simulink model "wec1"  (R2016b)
settings: Solver=ode45  StartTime=0  StopTime=1000  FixedStep=0.005  MaxStep=0.005  RelTol=1e-3
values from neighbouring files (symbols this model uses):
  arAdaptiveLawData = 1/2*zModelSimple.zModelPto.arFreq.*     zModelSimple.zModelPto.arMagnitude./     cos(zModelSimple.zModelPto.arPhase*pi/180+pi/2)    [IMPACT_Control.m]
  arControllerRampGain = [0,0,1,1]    [IMPACT_Control.m]
  arControllerRampTime = [0 rStartRampTime rStartRampTime+rRampTimeLength 8000]    [IMPACT_Control.m]
  arEkfInitialisation = zeros(1,11)    [IMPACT_Control.m]
  arFrequency = zModelSimple.zModelPto.arFreq    [IMPACT_Control.m]
  arFrequencyRange = zModelSimple.zModelPto.arFreq    [IMPACT_Control.m]
  arImpedance = 1./zModelSimple.zModelPto.arMagnitude./zModelSimple.zModelPto.arFreq    [IMPACT_Control.m]
  iAdaptiveDamping = 0    [wec1_IMPACT_Project.m]    (also in IMPACT_Control.m = handles.iAdaptiveDamping; wec2_IMPACT_Project.m; wec3_IMPACT_Project.m; wec4IMPACT_Project.m)
  iControlType = 1    [wec1_IMPACT_Project.m]    (also in IMPACT_Control.m = handles.iControlType; wec2_IMPACT_Project.m; wec3_IMPACT_Project.m; wec4IMPACT_Project.m = 2)
  iPtoPositionConstraint = 0    [wec1_IMPACT_Project.m]    (also in IMPACT_Control.m = handles.iPtoPositionConstraint; wec2_IMPACT_Project.m = 1; wec3_IMPACT_Project.m = 1; wec4IMPACT_Project.m = 1)
  iSensorNoise = 0    [IMPACT_Control.m]
  m = m+1    (= 2)    [checkParamFile.m]
  rAccelerationGainPosLim = 9.4530e+06    (= 9453000)    [wec1AdditionalParams.m]    (also in wec2AdditionalParams.m = 4513300)
  rBalancingForce = -(rFloaterVolume*rDENSITY - rFloaterMass)*rGRAVITY    [IMPACT_Control.m]
  rBuoyancyGainPosLim = 3.1355e+06    (= 3135500)    [wec1AdditionalParams.m]    (also in wec2AdditionalParams.m = 7.4216)
  rCogFloater = -18    [wec1_IMPACT_Model.m]    (also in paramInitial.m = get( handles.edit_rCogFloater, 'String' ); wec2_IMPACT_Model.m = -8.5; wec3_IMPACT_Model.m = -0.7; wec3_IMPACT_Model2.m = -0.7)
  rDampingGainPosLim = 2.0369e+05    (= 203690)    [wec1AdditionalParams.m]    (also in wec2AdditionalParams.m = 11575)
  rDisplacementLimit = 10.000000    (= 10)    [wec1_IMPACT_Project.m]    (also in IMPACT_Control.m = getValue(handles.edit_displacementLimit); wec2_IMPACT_Project.m; wec3_IMPACT_Project.m = 3; wec4IMPACT_Project.m)
  rGainForAntiWIndUp = tfControllerDiscrete.rGain    [IMPACT_Control.m]
  rMaxForcePto = 1000000000000000.000000    (= 1e+15)    [wec1_IMPACT_Project.m]    (also in IMPACT_Control.m = getValue(handles.edit_maxForcePto); wec2_IMPACT_Project.m; wec3_IMPACT_Project.m = 1000000000; wec4IMPACT_Project.m = 300000000)
  rMinForcePto = -1000000000000000.000000    (= -1e+15)    [wec1_IMPACT_Project.m]    (also in IMPACT_Control.m = getValue(handles.edit_minForcePto); wec2_IMPACT_Project.m; wec3_IMPACT_Project.m = -1000000000; wec4IMPACT_Project.m = -300000000)
  rOutputSampleTime = 0.010000    (= 0.01)    [wec1_IMPACT_Project.m]    (also in IMPACT_Control.m = getValue(handles.edit_outputSampleTime); wec2_IMPACT_Project.m; wec3_IMPACT_Project.m; wec4IMPACT_Project.m)
  rPassiveDampingGain = -214018.153700    (= -214018.1537)    [wec1_IMPACT_Project.m]    (also in IMPACT_Control.m = getValue(handles.edit_gainPLD); wec2_IMPACT_Project.m = -1948070; wec3_IMPACT_Project.m = -519390; wec4IMPACT_Project.m = -604830)
  rPositionLimitRatio = 10    [wec1AdditionalParams.m]    (also in wec2AdditionalParams.m)
  rUpperFrequencyLimit = EKFFloater.upperFreq    [IMPACT_Control.m]
  s = tf('s')    [wec1_IMPACT_Model.m]    (also in IMPACT_Control.m; wec2_IMPACT_Model.m; wec3_IMPACT_Model.m; wec3_IMPACT_Model2.m)
  simu = simulationClass()    [wecSimInputFile.m]
  Z = magPhaseToComplex(zModelTf)    [IMPACT_Control.m]
undefined symbols (not defined in the file or in its folder): arExcForceFloaterDen, arExcForceFloaterNum, body, N, pto, rAccelerationGainFloater, rBuoyancyGainFloater, rDampingGainFloater, X, Y
libraries: nesl_utility x9, sm_lib x5, simulink x3, WECSim_Lib x2

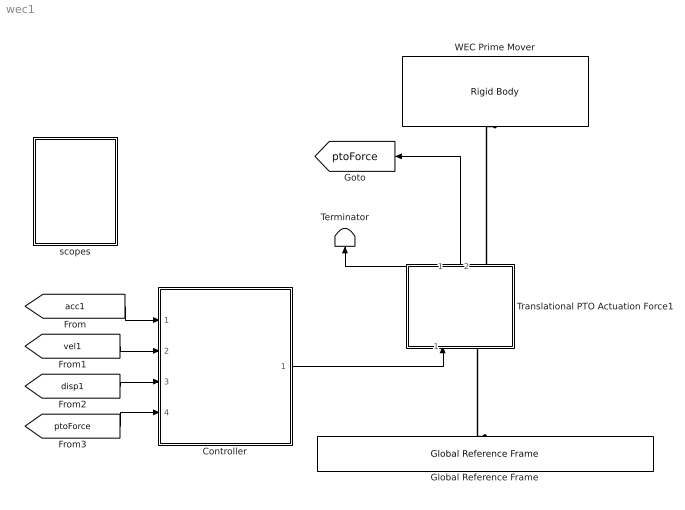
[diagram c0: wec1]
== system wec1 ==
  Controller : Subsystem
  Global Reference Frame : WECSim_Lib/Frames/Global Reference Frame  waves=waves  simu=simu
  Terminator : Terminator
  Translational PTO Actuation Force1 : Subsystem  AncestorBlock=WECSim_Lib/PTOs/Translational PTO Actuation Force
  WEC Prime Mover : WECSim_Lib/Body Elements/Rigid Body  body=body(1)
  scopes : Subsystem
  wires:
  Translational PTO Actuation Force1/2(ptoForce) -> [ptoForce]
  Controller/1(forceDemand) -> Translational PTO Actuation Force1/1(Force)
  Translational PTO Actuation Force1/1(Response) -> Terminator/1
  [disp1] -> Controller/3(Floater displacement)
  [vel1] -> Controller/2(Floater velocity)
  [acc1] -> Controller/1(Floater acceleration)
  [ptoForce] -> Controller/4(PTO Force)
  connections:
  Translational PTO Actuation Force1/RConn1 -- WEC Prime Mover/RConn1
  Translational PTO Actuation Force1/LConn1 -- Global Reference Frame/RConn1

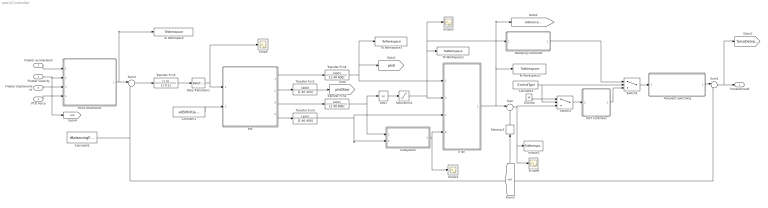
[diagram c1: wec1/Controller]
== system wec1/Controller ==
  Floater acceleration : Inport
  Floater velocity : Inport  Port=2
  Floater displacement : Inport  Port=3
  PTO Force : Inport  Port=4
  Abs1 : Abs
  Constant1 : Constant  Value=arEkfInitialisation
  Constant3 : Constant  Value=iControlType
  Constant5 : Constant  Value=rBalancingForce
  Damping Controller : Subsystem
  EKF : MATLAB Function  TreatAsAtomicUnit=on
  "Force estimation " : Subsystem
  Ground : Ground
  OVT Controller : Subsystem
  Rate Transition1 : RateTransition  OutPortSampleTimeMultiple=0.01  OutPortSampleTime=rKalmanFilterSampleTime
  Saturation1 : Saturate  UpperLimit=rUpperFrequencyLimit  LowerLimit=0  LinearizeAsGain=off
  Scope{,1..2,8} (4 alike) : Scope
  Selector2 : Selector  InputPortWidth=6  IndexOptions=Index vector (dialog)  Indices=3  OutputSizes=1
  Subsystem : Subsystem
  Sum : Sum  Inputs=|+-
  Sum1 : Sum  Inputs=|++
  Sum2 : Sum  Inputs=|++
  Switch1 : Switch  Threshold=2
  Switch2 : Switch  Threshold=2
  To Workspace : ToWorkspace  VariableName=arEstimatedExcitationForce1  SampleTime=rOutputSampleTime
  To Workspace1 : ToWorkspace  VariableName=arEkfFrequency  SampleTime=rOutputSampleTime
  To Workspace2 : ToWorkspace  VariableName=arReferenceVelocity  SampleTime=rOutputSampleTime
  To Workspace3 : ToWorkspace  VariableName=arEkfAmplitude  SampleTime=rOutputSampleTime
  Transfer Fcn{1..2,4..5} (4 alike) : TransferFcn  Numerator=[400]  Denominator=[1 40 400]
  Transfer Fcn3 : TransferFcn  Numerator=[1 0]  Denominator=[1 0.1]
  Transient Switching : Subsystem
  "V ref " : Subsystem
  output1 : ToWorkspace  VariableName=arError  SampleTime=rOutputSampleTime
  forceDemand : Outport
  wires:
  Damping Controller/1(forceDemand) -> Switch1/1
  Sum/1 -> output1/1, Scope8/1, Switch2/3
  Selector2/1 -> Sum/2
  "V ref "/1(referenceVelocity) -> To Workspace2/1, [referenceVelocity], Sum/1
  [vel1] -> Selector2/1
  OVT Controller/1(forceDemand) -> Switch1/3
  Saturation1/1 -> Scope2/1, Damping Controller/1(ekfFrequency), To Workspace1/1, "V ref "/2(ekfFrequency)
  EKF/4(rAmplitudeOutput) -> Transfer Fcn5/1
  EKF/3(rFrequencyOutput) -> Transfer Fcn2/1
  EKF/1(rPhi0Output) -> Transfer Fcn4/1
  Rate Transition1/1 -> Scope/1, EKF/1(rEstimatedExcitationForce)
  EKF/2(rPhi0StarOutput) -> Transfer Fcn1/1
  Abs1/1 -> Saturation1/1
  Switch1/1 -> Transient Switching/1(forceDemandIn)
  Sum1/1 -> [forceDemand], forceDemand/1
  Constant5/1 -> Sum1/2, Sum2/2
  Transfer Fcn3/1 -> Rate Transition1/1
  Constant1/1 -> EKF/2(arEkfInitialisation)
  "Force estimation "/1(estimatedExcitationForce) -> To Workspace/1, Sum2/1
  Switch2/1 -> OVT Controller/1(error)
  Transient Switching/1(forceDemandOut) -> Sum1/1
  Sum2/1 -> Transfer Fcn3/1
  Transfer Fcn4/1 -> "V ref "/1(phiOut), To Workspace3/1, [phi0]
  Transfer Fcn1/1 -> [phi0Star]
  Transfer Fcn2/1 -> Abs1/1, Subsystem/1(frequency)
  Transfer Fcn5/1 -> Subsystem/2(excitationForce), "V ref "/3(ekfAmplitude)
  Subsystem/1(displacementLimit) -> Scope1/1, "V ref "/4(limit)
  Ground/1 -> Switch2/1
  Floater acceleration/1 -> "Force estimation "/1(Acceleration)
  Floater displacement/1 -> "Force estimation "/3(Position)
  Floater velocity/1 -> [vel1], "Force estimation "/2(Velocity)
  PTO Force/1 -> "Force estimation "/4(PTO Force)
  Constant3/1 -> Switch2/2, Switch1/2

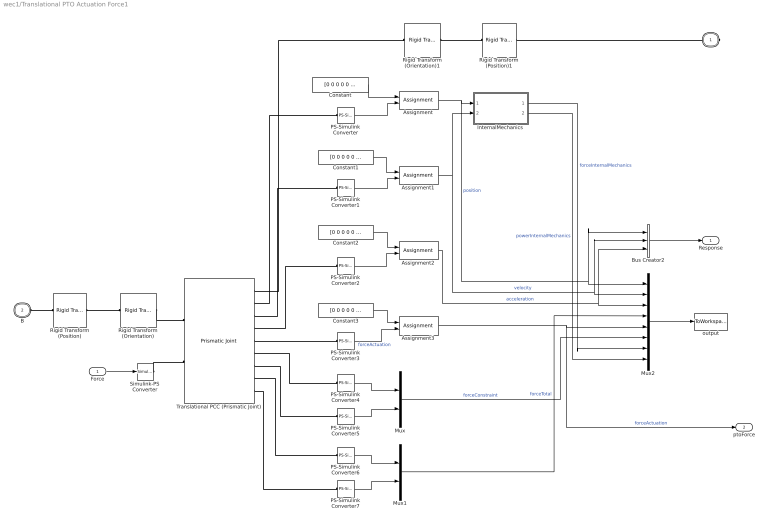
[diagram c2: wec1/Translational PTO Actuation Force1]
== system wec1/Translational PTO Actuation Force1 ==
  Force : Inport
  Assignment{,1..3} (4 alike) : Assignment  IndexOptions=Index vector (dialog)  Indices=3  OutputSizes=1
  Bus Creator2 : BusCreator  Inputs=3
  Constant{,1..3} (4 alike) : Constant  Value=[0 0 0 0 0 0]
  InternalMechanics : Subsystem
  Mux : Mux  Inputs=2
  Mux1 : Mux  Inputs=2
  Mux2 : Mux  Inputs=8
  PS-Simulink Converter{,1..7} (8 alike) : nesl_utility/PS-Simulink Converter  PhysicalDomain=network_engine_domain  SubClassName=ps_output  LeftPortType=input  RightPortType=output  PseudoPeriodic=off  Frequencies=[]  Unit=1  AffineConversion=off
  Rigid Transform (Position) : sm_lib/Frames and Transforms/Rigid Transform  TranslationMethod=Cartesian  TranslationStandardOffset=0  TranslationLengthUnit=m  TranslationStandardAxis=+Z  TranslationCartesianOffset=pto.initDisp.initLinDisp + pto.loc  TranslationROffset=0  TranslationROffsetUnits=m  TranslationZOffset=0  TranslationZOffsetUnits=m  TranslationThetaOffset=0  TranslationThetaOffsetUnits=deg  RotationMethod=None  RotationAngleUnits=rad  RotationStandardAxis=+Y  RotationAngle=0  RotationArbitraryAxis=[0 1 0]  FollAlignAxisA=+X  BaseAlignAxisA=+Y  FollAlignAxisB=+Y  BaseAlignAxisB=+Z  RotationSequenceAxes=FollowerAxes  RotationSequence=XYX  RotationSequenceAngles=[0 0 0]  RotationSequenceAnglesUnits=deg  RotationMatrix=[1 0 0; 0 1 0; 0 0 1]
  Rigid Transform (Position)1 : sm_lib/Frames and Transforms/Rigid Transform  TranslationMethod=Cartesian  TranslationStandardOffset=0  TranslationLengthUnit=m  TranslationStandardAxis=+Z  TranslationCartesianOffset=pto.initDisp.initLinDisp + pto.loc  TranslationROffset=0  TranslationROffsetUnits=m  TranslationZOffset=0  TranslationZOffsetUnits=m  TranslationThetaOffset=0  TranslationThetaOffsetUnits=deg  RotationMethod=None  RotationAngleUnits=rad  RotationStandardAxis=+Y  RotationAngle=0  RotationArbitraryAxis=[0 1 0]  FollAlignAxisA=+X  BaseAlignAxisA=+Y  FollAlignAxisB=+Y  BaseAlignAxisB=+Z  RotationSequenceAxes=FollowerAxes  RotationSequence=XYX  RotationSequenceAngles=[0 0 0]  RotationSequenceAnglesUnits=deg  RotationMatrix=[1 0 0; 0 1 0; 0 0 1]
  Rigid Transform (Orientation) : sm_lib/Frames and Transforms/Rigid Transform  TranslationMethod=None  TranslationStandardOffset=0  TranslationLengthUnit=m  TranslationStandardAxis=+Z  TranslationCartesianOffset=0  TranslationROffset=0  TranslationROffsetUnits=m  TranslationZOffset=0  TranslationZOffsetUnits=m  TranslationThetaOffset=0  TranslationThetaOffsetUnits=deg  RotationMethod=RotationMatrix  RotationAngleUnits=rad  RotationStandardAxis=+Y  RotationAngle=0  RotationArbitraryAxis=[0 1 0]  FollAlignAxisA=+X  BaseAlignAxisA=+Y  FollAlignAxisB=+Y  BaseAlignAxisB=+Z  RotationSequenceAxes=FollowerAxes  RotationSequence=XYX  RotationSequenceAngles=[0 0 0]  RotationSequenceAnglesUnits=deg  RotationMatrix=pto.orientation.rotationMatrix
  Rigid Transform (Orientation)1 : sm_lib/Frames and Transforms/Rigid Transform  TranslationMethod=None  TranslationStandardOffset=0  TranslationLengthUnit=m  TranslationStandardAxis=+Z  TranslationCartesianOffset=0  TranslationROffset=0  TranslationROffsetUnits=m  TranslationZOffset=0  TranslationZOffsetUnits=m  TranslationThetaOffset=0  TranslationThetaOffsetUnits=deg  RotationMethod=RotationMatrix  RotationAngleUnits=rad  RotationStandardAxis=+Y  RotationAngle=0  RotationArbitraryAxis=[0 1 0]  FollAlignAxisA=+X  BaseAlignAxisA=+Y  FollAlignAxisB=+Y  BaseAlignAxisB=+Z  RotationSequenceAxes=FollowerAxes  RotationSequence=XYX  RotationSequenceAngles=[0 0 0]  RotationSequenceAnglesUnits=deg  RotationMatrix=pto.orientation.rotationMatrix
  Simulink-PS Converter : nesl_utility/Simulink-PS Converter  PhysicalDomain=network_engine_domain  SubClassName=ps_input  LeftPortType=input  RightPortType=output  PseudoPeriodic=off  Frequencies=[]  NoiseDistribution=none  NoiseParameters=[]  Unit=1  AffineConversion=off  InputFiltering=off  SimscapeFilterOrder=1  InputFilterTimeConstant=0.001  UdotUserProvided=1
  Translational PCC (Prismatic Joint) : sm_lib/Joints/Prismatic Joint  SenseConstraintForce=on  SenseConstraintForceX=off  SenseConstraintForceY=off  SenseConstraintForceZ=off  SenseConstraintTorque=on  SenseConstraintTorqueX=off  SenseConstraintTorqueY=off  SenseConstraintTorqueZ=off  SenseTotalForce=on  SenseTotalForceX=off  SenseTotalForceY=off  SenseTotalForceZ=off  SenseTotalTorque=on  SenseTotalTorqueX=off  SenseTotalTorqueY=off  SenseTotalTorqueZ=off  CompositeWrenchDir=BaseOnFollower  CompositeWrenchFrame=BaseFrame  EquilibriumPosition=0  EquilibriumPositionUnits=m  SpringStiffness=pto.k  SpringStiffnessUnits=N/m  DampingCoefficient=pto.c  DampingCoefficientUnits=N/(m/s)  TorqueActuationMode=InputTorque  MotionActuationMode=ComputedMotion  SensePosition=on  SenseVelocity=on  SenseAcceleration=on  SenseTorqueForce=on  PositionTargetSpecify=off  PositionTargetPriority=High  PositionTargetValue=0  PositionTargetValueUnits=m  VelocityTargetSpecify=off  VelocityTargetPriority=High  VelocityTargetValue=0  VelocityTargetValueUnits=m/s
  output : ToWorkspace  VariableName=pto1_out  SaveFormat=Structure With Time  SampleTime=-1
  F : PMIOPort  Port=1  Side=Right
  B : PMIOPort  Port=2  Side=Left
  Response : Outport
  ptoForce : Outport  Port=2
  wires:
  Bus Creator2/1 -> Response/1
  Assignment/1 -> Mux2/1, Bus Creator2/1, InternalMechanics/1(Position)  "position"
  Assignment1/1 -> Mux2/2, Bus Creator2/2, InternalMechanics/2(Velocity)  "velocity"
  Assignment2/1 -> Mux2/3, Bus Creator2/3  "acceleration"
  Force/1 -> Simulink-PS Converter/1
  Mux2/1 -> output/1
  Mux/1 -> Mux2/6  "forceConstraint"
  Mux1/1 -> Mux2/4  "forceTotal"
  PS-Simulink Converter4/1 -> Mux/1
  PS-Simulink Converter5/1 -> Mux/2
  PS-Simulink Converter6/1 -> Mux1/1
  PS-Simulink Converter7/1 -> Mux1/2
  Assignment3/1 -> ptoForce/1, Mux2/5  "forceActuation"
  Constant/1 -> Assignment/1
  PS-Simulink Converter/1 -> Assignment/2
  Constant1/1 -> Assignment1/1
  PS-Simulink Converter1/1 -> Assignment1/2
  Constant2/1 -> Assignment2/1
  PS-Simulink Converter2/1 -> Assignment2/2
  InternalMechanics/1(Force) -> Mux2/7  "forceInternalMechanics"
  InternalMechanics/2(Power) -> Mux2/8  "powerInternalMechanics"
  Constant3/1 -> Assignment3/1
  PS-Simulink Converter3/1 -> Assignment3/2  "forceActuation"
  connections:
  Rigid Transform (Position)/RConn1 -- Rigid Transform (Orientation)/LConn1
  Rigid Transform (Position)1/RConn1 -- Rigid Transform (Orientation)1/LConn1
  Simulink-PS Converter/RConn1 -- Translational PCC (Prismatic Joint)/LConn2
  Rigid Transform (Orientation)/RConn1 -- Translational PCC (Prismatic Joint)/LConn1
  Rigid Transform (Position)/LConn1 -- B/RConn1
  Translational PCC (Prismatic Joint)/RConn5 -- PS-Simulink Converter3/LConn1
  Translational PCC (Prismatic Joint)/RConn9 -- PS-Simulink Converter7/LConn1
  Rigid Transform (Orientation)1/RConn1 -- Translational PCC (Prismatic Joint)/RConn1
  Translational PCC (Prismatic Joint)/RConn4 -- PS-Simulink Converter2/LConn1
  Translational PCC (Prismatic Joint)/RConn7 -- PS-Simulink Converter5/LConn1
  Translational PCC (Prismatic Joint)/RConn3 -- PS-Simulink Converter1/LConn1
  Rigid Transform (Position)1/LConn1 -- F/RConn1
  Translational PCC (Prismatic Joint)/RConn8 -- PS-Simulink Converter6/LConn1
  Translational PCC (Prismatic Joint)/RConn2 -- PS-Simulink Converter/LConn1
  Translational PCC (Prismatic Joint)/RConn6 -- PS-Simulink Converter4/LConn1

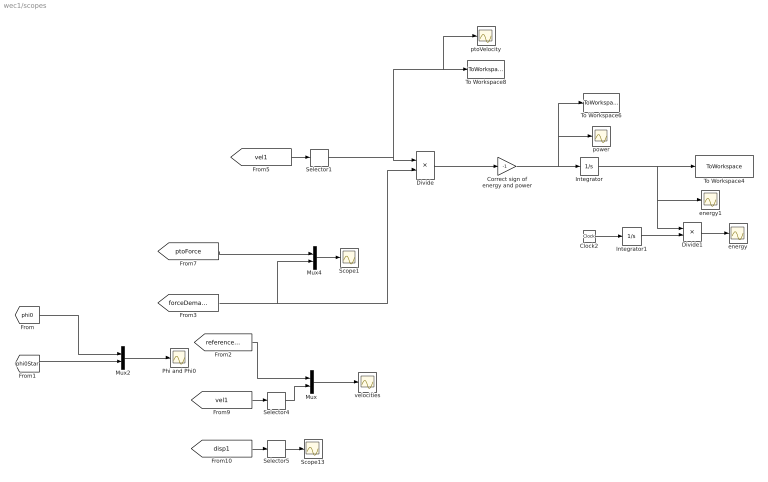
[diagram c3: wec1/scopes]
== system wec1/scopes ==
  Clock2 : Clock
  Correct sign of energy and power : Gain  Gain=-1
  Divide : Product  Inputs=**
  Divide1 : Product  Inputs=*/
  Integrator : Integrator
  Integrator1 : Integrator
  Mux : Mux  Inputs=2
  Mux2 : Mux  Inputs=2
  Mux4 : Mux  Inputs=2
  Phi and Phi0 : Scope
  Scope1 : Scope
  Scope13 : Scope
  Selector1 : Selector  InputPortWidth=6  IndexOptions=Index vector (dialog)  Indices=3  OutputSizes=1
  Selector4 : Selector  InputPortWidth=6  IndexOptions=Index vector (dialog)  Indices=3  OutputSizes=1
  Selector5 : Selector  InputPortWidth=6  IndexOptions=Index vector (dialog)  Indices=3  OutputSizes=1
  To Workspace4 : ToWorkspace  VariableName=arWecEnergy  SampleTime=rOutputSampleTime
  To Workspace6 : ToWorkspace  VariableName=arWecPower  SampleTime=rOutputSampleTime
  To Workspace8 : ToWorkspace  VariableName=arPtoVelocity  SampleTime=rOutputSampleTime
  energy : Scope
  energy1 : Scope
  power : Scope
  ptoVelocity : Scope
  velocities : Scope
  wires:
  [vel1] -> Selector4/1
  Mux/1 -> velocities/1
  Selector5/1 -> Scope13/1
  [phi0] -> Mux2/1
  Mux2/1 -> Phi and Phi0/1
  Mux4/1 -> Scope1/1
  Selector4/1 -> Mux/2
  [disp1] -> Selector5/1
  [referenceVelocity] -> Mux/1
  [forceDemand] -> Mux4/2, Divide/2
  Clock2/1 -> Integrator1/1
  Divide1/1 -> energy/1
  Integrator1/1 -> Divide1/2
  Integrator/1 -> To Workspace4/1, energy1/1, Divide1/1
  Divide/1 -> Correct sign of energy and power/1
  Selector1/1 -> Divide/1, ptoVelocity/1, To Workspace8/1
  [vel1] -> Selector1/1
  [phi0Star] -> Mux2/2
  Correct sign of energy and power/1 -> To Workspace6/1, power/1, Integrator/1
  [ptoForce] -> Mux4/1

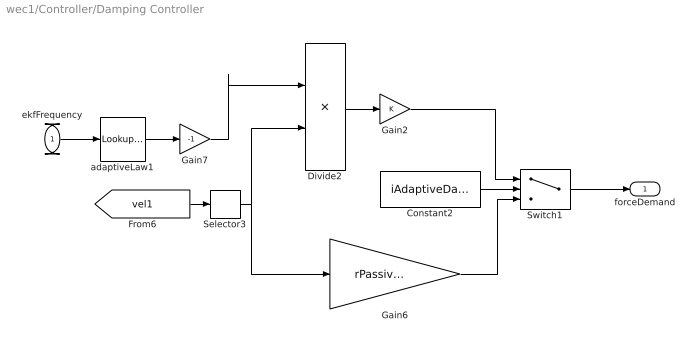
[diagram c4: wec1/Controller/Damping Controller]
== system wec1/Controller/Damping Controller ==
  ekfFrequency : Inport
  Constant2 : Constant  Value=iAdaptiveDamping
  Divide2 : Product  Inputs=**
  Gain2 : Gain
  Gain6 : Gain  Gain=rPassiveDampingGain
  Gain7 : Gain  Gain=-1
  Selector3 : Selector  InputPortWidth=6  IndexOptions=Index vector (dialog)  Indices=3  OutputSizes=1
  Switch1 : Switch  Criteria=u2 > Threshold
  adaptiveLaw1 : Lookup_n-D  NumberOfTableDimensions=1  BreakpointsForDimension1=arFrequency  Table=arImpedance  InternalRulePriority=Speed  RndMeth=Simplest
  forceDemand : Outport
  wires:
  Gain2/1 -> Switch1/1
  ekfFrequency/1 -> adaptiveLaw1/1
  adaptiveLaw1/1 -> Gain7/1
  Constant2/1 -> Switch1/2
  Switch1/1 -> forceDemand/1
  Gain7/1 -> Divide2/1
  Selector3/1 -> Divide2/2, Gain6/1
  [vel1] -> Selector3/1
  Divide2/1 -> Gain2/1
  Gain6/1 -> Switch1/3

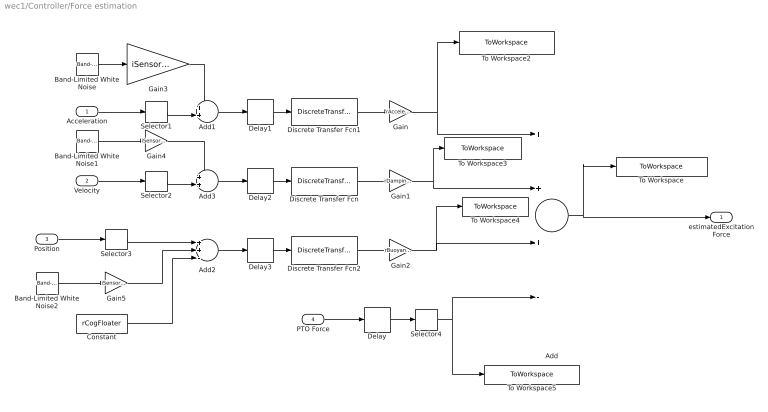
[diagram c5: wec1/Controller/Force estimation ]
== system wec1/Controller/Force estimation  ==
  Acceleration : Inport
  Velocity : Inport  Port=2
  Position : Inport  Port=3
  PTO Force : Inport  Port=4
  Add : Sum  Inputs=+++-
  Add1 : Sum  Inputs=++|
  Add2 : Sum  Inputs=++-
  Add3 : Sum  Inputs=++|
  Band-Limited White Noise : simulink/Sources/Band-Limited White Noise  Cov=rAccNoisePower  Ts=simu.dt  seed=[23341]
  Band-Limited White Noise1 : simulink/Sources/Band-Limited White Noise  Cov=rVelNoisePower  Ts=simu.dt  seed=[23341]
  Band-Limited White Noise2 : simulink/Sources/Band-Limited White Noise  Cov=rPosNoisePower  Ts=simu.dt  seed=[23341]
  Constant : Constant  Value=rCogFloater
  Delay{,1..3} (4 alike) : Delay  DelayLength=1  SampleTime=0.01
  Discrete Transfer Fcn : DiscreteTransferFcn  Numerator=arExcForceFloaterNum  Denominator=arExcForceFloaterDen  SampleTime=0.01
  Discrete Transfer Fcn1 : DiscreteTransferFcn  Numerator=arExcForceFloaterNum  Denominator=arExcForceFloaterDen  SampleTime=0.01
  Discrete Transfer Fcn2 : DiscreteTransferFcn  Numerator=arExcForceFloaterNum  Denominator=arExcForceFloaterDen  SampleTime=0.01
  Gain : Gain  Gain=rAccelerationGainFloater
  Gain1 : Gain  Gain=rDampingGainFloater
  Gain2 : Gain  Gain=rBuoyancyGainFloater
  Gain3 : Gain  Gain=iSensorNoise
  Gain4 : Gain  Gain=iSensorNoise
  Gain5 : Gain  Gain=iSensorNoise
  Selector{1..4} (4 alike) : Selector  InputPortWidth=6  IndexOptions=Index vector (dialog)  Indices=3  OutputSizes=1
  To Workspace : ToWorkspace  VariableName=arEstimatedExcitationForce  SampleTime=rOutputSampleTime
  To Workspace2 : ToWorkspace  VariableName=arAccelerationComponent  SampleTime=rOutputSampleTime
  To Workspace3 : ToWorkspace  VariableName=arVelocityComponent  SampleTime=rOutputSampleTime
  To Workspace4 : ToWorkspace  VariableName=arPositionComponent  SampleTime=rOutputSampleTime
  To Workspace5 : ToWorkspace  VariableName=arPtoForceMeasurement  SampleTime=rOutputSampleTime
  estimatedExcitationForce : Outport
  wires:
  Selector1/1 -> Add1/2
  Band-Limited White Noise/1 -> Gain3/1
  Acceleration/1 -> Selector1/1
  Gain5/1 -> Add2/2
  Add2/1 -> Delay3/1
  Position/1 -> Selector3/1
  Add/1 -> To Workspace/1, estimatedExcitationForce/1
  Gain2/1 -> To Workspace4/1, Add/3
  Gain/1 -> To Workspace2/1, Add/1
  Constant/1 -> Add2/3
  Gain4/1 -> Add3/1
  Velocity/1 -> Selector2/1
  Gain3/1 -> Add1/1
  Selector2/1 -> Add3/2
  Add1/1 -> Delay1/1
  Selector3/1 -> Add2/1
  Band-Limited White Noise1/1 -> Gain4/1
  Band-Limited White Noise2/1 -> Gain5/1
  Selector4/1 -> To Workspace5/1, Add/4
  Delay/1 -> Selector4/1
  Delay1/1 -> Discrete Transfer Fcn1/1
  Delay2/1 -> Discrete Transfer Fcn/1
  Delay3/1 -> Discrete Transfer Fcn2/1
  Gain1/1 -> Add/2, To Workspace3/1
  Add3/1 -> Delay2/1
  Discrete Transfer Fcn1/1 -> Gain/1
  Discrete Transfer Fcn/1 -> Gain1/1
  Discrete Transfer Fcn2/1 -> Gain2/1
  PTO Force/1 -> Delay/1

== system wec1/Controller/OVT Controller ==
  error : Inport
  Anti wind-up controller : Subsystem
  forceDemand : Outport
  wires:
  error/1 -> Anti wind-up controller/1(error)
  Anti wind-up controller/1(Out1) -> forceDemand/1

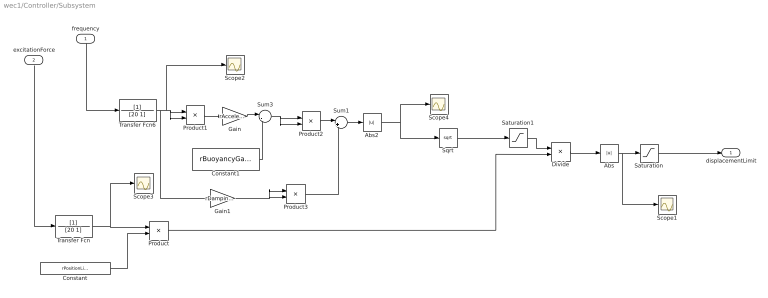
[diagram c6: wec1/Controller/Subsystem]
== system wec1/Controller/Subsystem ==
  frequency : Inport
  excitationForce : Inport  Port=2
  Abs : Abs
  Abs2 : Abs
  Constant : Constant  Value=rPositionLimitRatio
  Constant1 : Constant  Value=rBuoyancyGainPosLim
  Divide : Product  Inputs=/*
  Gain : Gain  Gain=rAccelerationGainPosLim
  Gain1 : Gain  Gain=rDampingGainPosLim
  Product{,1..3} (4 alike) : Product
  Saturation : Saturate  UpperLimit=10  LowerLimit=0
  Saturation1 : Saturate  UpperLimit=inf  LowerLimit=0.0001
  Scope{1..4} (4 alike) : Scope
  Sqrt : Sqrt
  Sum1 : Sum  Inputs=|++
  Sum3 : Sum  Inputs=|-+
  Transfer Fcn : TransferFcn  Denominator=[20 1]
  Transfer Fcn6 : TransferFcn  Denominator=[20 1]
  displacementLimit : Outport
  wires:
  Product1/1 -> Gain/1
  Gain/1 -> Sum3/1
  Transfer Fcn6/1 -> Gain1/1, Scope2/1, Product1/2, Product1/1
  Constant1/1 -> Sum3/2
  Product/1 -> Divide/2
  Constant/1 -> Product/2
  Transfer Fcn/1 -> Scope3/1, Product/1
  frequency/1 -> Transfer Fcn6/1
  excitationForce/1 -> Transfer Fcn/1
  Divide/1 -> Abs/1
  Sum3/1 -> Product2/1, Product2/2
  Abs/1 -> Scope1/1, Saturation/1
  Saturation/1 -> displacementLimit/1
  Saturation1/1 -> Divide/1
  Abs2/1 -> Scope4/1, Sqrt/1
  Product2/1 -> Sum1/1
  Gain1/1 -> Product3/1, Product3/2
  Product3/1 -> Sum1/2
  Sum1/1 -> Abs2/1
  Sqrt/1 -> Saturation1/1

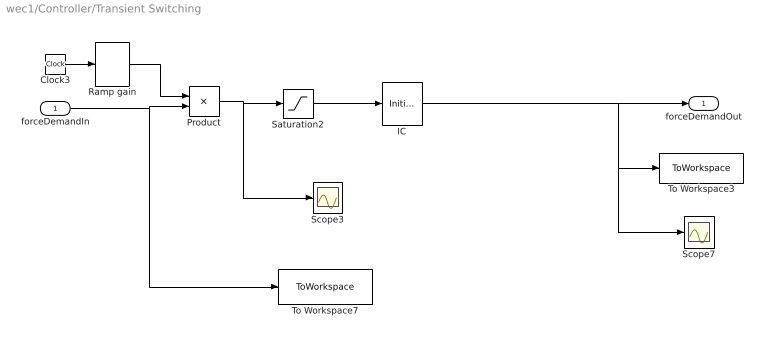
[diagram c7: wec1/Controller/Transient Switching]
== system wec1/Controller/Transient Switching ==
  forceDemandIn : Inport
  Clock3 : Clock
  IC : InitialCondition  Value=0
  Product : Product
  Ramp gain : Lookup_n-D  NumberOfTableDimensions=1  BreakpointsForDimension1=arControllerRampTime  Table=arControllerRampGain  InternalRulePriority=Speed  RndMeth=Simplest
  Saturation2 : Saturate  UpperLimit=rMaxForcePto  LowerLimit=rMinForcePto
  Scope3 : Scope
  Scope7 : Scope
  To Workspace3 : ToWorkspace  VariableName=arForceDemand  SampleTime=rOutputSampleTime
  To Workspace7 : ToWorkspace  VariableName=arForceDemandIn  SampleTime=rOutputSampleTime
  forceDemandOut : Outport
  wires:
  Clock3/1 -> Ramp gain/1
  Saturation2/1 -> IC/1
  Product/1 -> Saturation2/1, Scope3/1
  forceDemandIn/1 -> Product/2, To Workspace7/1
  IC/1 -> To Workspace3/1, Scope7/1, forceDemandOut/1
  Ramp gain/1 -> Product/1

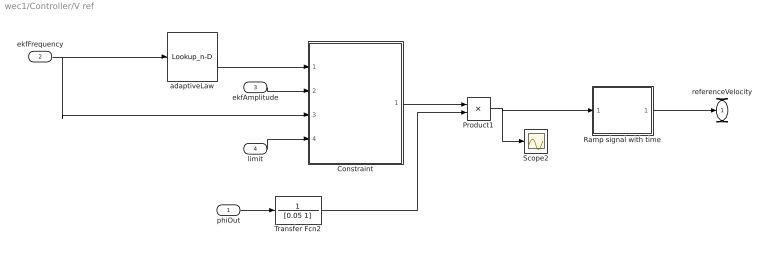
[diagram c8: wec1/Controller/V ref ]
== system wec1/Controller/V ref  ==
  phiOut : Inport
  ekfFrequency : Inport  Port=2
  ekfAmplitude : Inport  Port=3
  limit : Inport  Port=4
  Constraint : Subsystem
  Product1 : Product
  Ramp signal with time : Subsystem
  Scope2 : Scope
  Transfer Fcn2 : TransferFcn  Numerator=1  Denominator=[0.05 1]
  adaptiveLaw : Lookup_n-D  NumberOfTableDimensions=1  BreakpointsForDimension1=arFrequencyRange  Table=arAdaptiveLawData  InternalRulePriority=Speed  RndMeth=Simplest
  referenceVelocity : Outport
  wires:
  Constraint/1(referenceVelocity) -> Product1/1
  phiOut/1 -> Transfer Fcn2/1
  adaptiveLaw/1 -> Constraint/1(1/2B)
  ekfFrequency/1 -> Constraint/3(ekfFrequency), adaptiveLaw/1
  Transfer Fcn2/1 -> Product1/2
  ekfAmplitude/1 -> Constraint/2(Amp)
  Product1/1 -> Ramp signal with time/1(In1), Scope2/1
  limit/1 -> Constraint/4(limit)
  Ramp signal with time/1(Out1) -> referenceVelocity/1

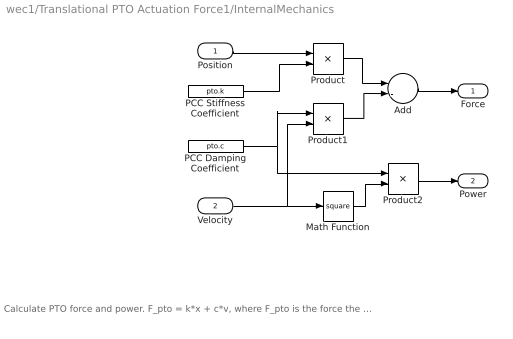
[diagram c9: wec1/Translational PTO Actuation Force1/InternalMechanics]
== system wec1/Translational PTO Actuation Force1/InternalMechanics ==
  note: Calculate PTO force and power. F_pto = k*x + c*v, where F_pto is the force the PTO applies to the body (at the PTO location), x and v are the joint position and velocity. The power extracted is P = c * v^2
  Position : Inport
  Velocity : Inport  Port=2
  Add : Sum  Inputs=--
  Math Function : Math  Operator=square
  PCC Damping Coefficient : Constant  Value=pto.c
  PCC Stiffness Coefficient : Constant  Value=pto.k
  Product : Product  Inputs=**
  Product1 : Product  Inputs=**
  Product2 : Product  Inputs=**
  Force : Outport
  Power : Outport  Port=2
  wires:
  PCC Damping Coefficient/1 -> Product2/1, Product1/1
  Product2/1 -> Power/1
  Velocity/1 -> Math Function/1, Product1/2
  PCC Stiffness Coefficient/1 -> Product/2
  Position/1 -> Product/1
  Add/1 -> Force/1
  Math Function/1 -> Product2/2
  Product/1 -> Add/1
  Product1/1 -> Add/2

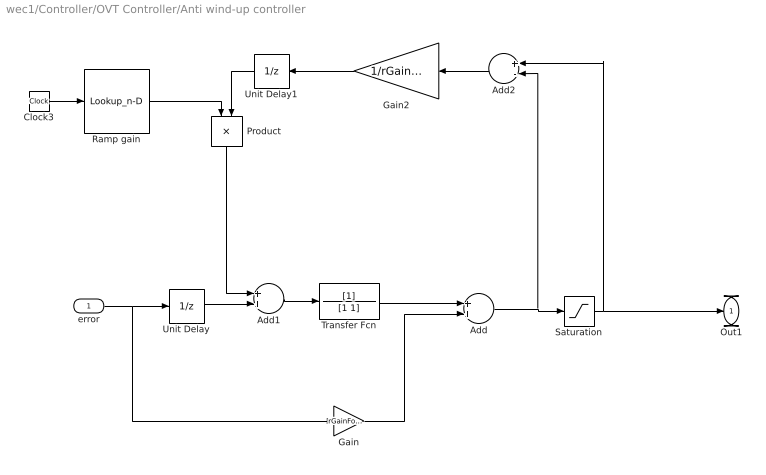
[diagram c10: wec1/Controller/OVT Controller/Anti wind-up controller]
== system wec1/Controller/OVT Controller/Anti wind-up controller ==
  error : Inport
  Add : Sum
  Add1 : Sum
  Add2 : Sum  Inputs=+-
  Clock3 : Clock
  Gain : Gain  Gain=rGainForAntiWIndUp
  Gain2 : Gain  Gain=1/rGainForAntiWIndUp
  Product : Product
  Ramp gain : Lookup_n-D  NumberOfTableDimensions=1  BreakpointsForDimension1=arControllerRampTime  Table=arControllerRampGain  InternalRulePriority=Speed  RndMeth=Simplest
  Saturation : Saturate  UpperLimit=rMaxForcePto  LowerLimit=rMinForcePto
  Transfer Fcn : TransferFcn  Denominator=[1 1]
  Unit Delay : UnitDelay  SampleTime=0.01
  Unit Delay1 : UnitDelay  SampleTime=0.01
  Out1 : Outport
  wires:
  Add/1 -> Saturation/1, Add2/2
  Gain/1 -> Add/2
  Unit Delay/1 -> Add1/2
  Gain2/1 -> Unit Delay1/1
  error/1 -> Gain/1, Unit Delay/1
  Add2/1 -> Gain2/1
  Add1/1 -> Transfer Fcn/1
  Clock3/1 -> Ramp gain/1
  Ramp gain/1 -> Product/1
  Product/1 -> Add1/1
  Unit Delay1/1 -> Product/2
  Transfer Fcn/1 -> Add/1
  Saturation/1 -> Add2/1, Out1/1

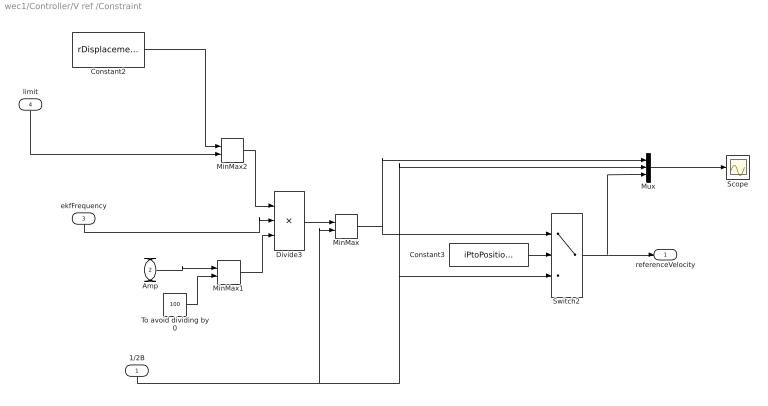
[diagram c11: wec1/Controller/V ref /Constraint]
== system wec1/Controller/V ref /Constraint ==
  1/2B : Inport
  Amp : Inport  Port=2
  ekfFrequency : Inport  Port=3
  limit : Inport  Port=4
  Constant2 : Constant  Value=rDisplacementLimit
  Constant3 : Constant  Value=iPtoPositionConstraint
  Divide3 : Product  Inputs=**/
  MinMax : MinMax  Inputs=2
  MinMax1 : MinMax  Function=max  Inputs=2
  MinMax2 : MinMax  Inputs=2
  Mux : Mux  Inputs=3
  Scope : Scope
  Switch2 : Switch  Criteria=u2 > Threshold
  To avoid dividing by 0 : Constant  Value=100
  referenceVelocity : Outport
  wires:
  MinMax/1 -> Mux/1, Switch2/1
  ekfFrequency/1 -> Divide3/2
  limit/1 -> MinMax2/2
  MinMax1/1 -> Divide3/3
  Divide3/1 -> MinMax/1
  To avoid dividing by 0/1 -> MinMax1/2
  Amp/1 -> MinMax1/1
  1/2B/1 -> MinMax/2, Mux/2, Switch2/3
  Constant3/1 -> Switch2/2
  Switch2/1 -> Mux/3, referenceVelocity/1
  Mux/1 -> Scope/1
  Constant2/1 -> MinMax2/1
  MinMax2/1 -> Divide3/1

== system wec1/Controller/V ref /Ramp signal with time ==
  In1 : Inport
  Clock3 : Clock
  Divide4 : Product  Inputs=**
  Ramp gain : Lookup_n-D  NumberOfTableDimensions=1  BreakpointsForDimension1=arControllerRampTime  Table=arControllerRampGain  InternalRulePriority=Speed  RndMeth=Simplest
  Out1 : Outport
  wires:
  Ramp gain/1 -> Divide4/1
  Clock3/1 -> Ramp gain/1
  Divide4/1 -> Out1/1
  In1/1 -> Divide4/2

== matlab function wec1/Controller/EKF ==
function [rPhi0Output,rPhi0StarOutput,rFrequencyOutput, rAmplitudeOutput]...
    = kalmanFilter(rEstimatedExcitationForce,arEkfInitialisation)
%%%%%%%%%%%%%%%%%%%%%%%%%%%%%%%%%%%%%%%%%%%%%%%%%%%%%%%%%%%%%%%%%%%%%%%%%
%%%                     Extended Kalman Filter                        %%%

%-----------------------------
% State equations
% X[n+1] = A*X[n] + B*U[n] + v
% Output equation
% Y[n] = C*X[n] + e
%-----------------------------
% n = Nº States
% m = Nº of inputs
% p = Nº of outputs
%
% See the IMPACT Deliverable 4 report for more detail on derivation of the
% Extended Kalman Filter
%
%%%%%%%%%%%%%%%%%%%%%%%%%%%%%%%%%%%%%%%%%%%%%%%%%%%%%%%%%%%%%%%%%%%%%%%%%

% Matrices of the system: A, B, C

persistent A B C P_k_k R1 R2 X_k_k bInit rFrequency rTimeStep rPhi0 rPhi0Star

% On the first step bInit is empty and so the initialisation can run

if isempty(bInit)
    
    bInit = 1;
    rFrequency = arEkfInitialisation(1);%0.5;
    rPhi0 = arEkfInitialisation(2);%1e5;
    rPhi0Star = arEkfInitialisation(3);%0;
    rTimeStep = arEkfInitialisation(4);
    
    A = zeros(3);
    A(1,:) = [cos(rFrequency*rTimeStep), sin(rFrequency*rTimeStep),...
        (-sin(rFrequency*rTimeStep)*rPhi0+cos(rFrequency*rTimeStep)*rPhi0Star)*rTimeStep];
    A(2,:) = [-sin(rFrequency*rTimeStep), cos(rFrequency*rTimeStep),...
        (-cos(rFrequency*rTimeStep)*rPhi0-sin(rFrequency*rTimeStep)*rPhi0Star)*rTimeStep];
    A(3,3) = 1;
    
    B = ones(3,1);
    C = zeros(1,3);
    C(1)=1;
    
%    Process noise covariance matrix
    R1 = [arEkfInitialisation(5),0,0;...
        0,arEkfInitialisation(6),0;...
        0,0,arEkfInitialisation(7)];

%   Measurement Noise covariance matrix
    R2 = arEkfInitialisation(8);

    % Initial values  
    P_k_k =  [arEkfInitialisation(9),0,0;...
        0,arEkfInitialisation(10),0;...
        0,0,arEkfInitialisation(11)];
    X_k_k = [rPhi0,rPhi0Star,rFrequency]';
end % End of initialisation

% No "input" for this EKF
U = 0;

% Time step consistent with simulation
rTimeStep = arEkfInitialisation(4);

% Define the A matrix as per deliverable 4 report
A(1,:) = [cos(rFrequency*rTimeStep) sin(rFrequency*rTimeStep) 0];
A(2,:) = [-sin(rFrequency*rTimeStep) cos(rFrequency*rTimeStep) 0];
A(3,3) = 1;


% Define the Jacobian as per deliverable 4 report - Note that for very
% small frequencies infinity must be avoided
JA = zeros(3);

if rFrequency<0.001 & rFrequency>=-0.001
    JA(1,:) = [cos(rFrequency*rTimeStep) sin(rFrequency*rTimeStep) rPhi0Star*rTimeStep-rPhi0*rFrequency*rTimeStep^2/2];
    JA(2,:) = [-sin(rFrequency*rTimeStep) cos(rFrequency*rTimeStep) -rPhi0*rTimeStep-rPhi0Star*rFrequency*rTimeStep^2/2];
    JA(3,3) = 1;
else
    JA(1,:) = [cos(rFrequency*rTimeStep) sin(rFrequency*rTimeStep) rPhi0Star*sin(rFrequency*rTimeStep)/rFrequency-rPhi0*(1-cos(rFrequency*rTimeStep))/rFrequency];
    JA(2,:) = [-sin(rFrequency*rTimeStep) cos(rFrequency*rTimeStep) -rPhi0*sin(rFrequency*rTimeStep)/rFrequency-rPhi0Star*(1-cos(rFrequency*rTimeStep))/rFrequency];
    JA(3,3) = 1;
end

% Define B and C Matrices
B = ones(3,1);
C = zeros(1,3);
C(1)=1;

% Kalman Filter
%---------------------------------
% Prediction
X_k1_k = A*X_k_k + B*U;

P_k1_k = JA*P_k_k*JA' + R1;

% Filter
Kf = P_k1_k*C'/(C*P_k1_k*C' + R2);
X_k1_k1 = X_k1_k + Kf*(rEstimatedExcitationForce-C*X_k1_k);
P_k1_k1 = P_k1_k - Kf*(C*P_k1_k*C'+R2)*Kf';


P_k_k = P_k1_k1; % for next cycle;
X_k_k = X_k1_k1; % for next cycle;

rFrequency = X_k_k(3);
rPhi0 = X_k_k(1);
rPhi0Star = X_k_k(2);

rFrequencyOutput = X_k_k(3);
rPhi0Output = X_k_k(1);
rPhi0StarOutput = X_k_k(2);
rAmplitudeOutput = sqrt(rPhi0.^2+rPhi0Star.^2);
